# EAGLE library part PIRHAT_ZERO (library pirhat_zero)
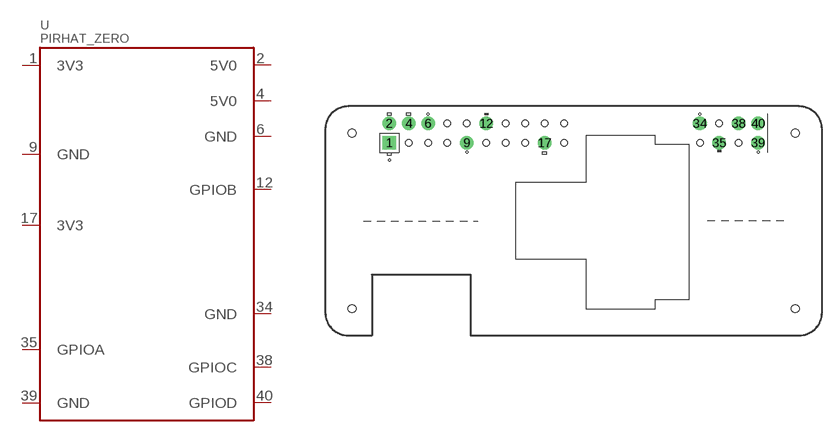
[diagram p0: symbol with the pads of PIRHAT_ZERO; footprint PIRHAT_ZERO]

Designator prefix -

## PIRHAT_ZERO  [PIRHAT_ZERO]
1  3V3  pwr
2  5V0  pwr
4  5V0  pwr
6  GND  sup
9  GND  sup
12  GPIOB
17  3V3  pwr
34  GND  sup
35  GPIOA
38  GPIOC
39  GND  sup
40  GPIOD

## Footprint PIRHAT_ZERO (pad centres in mm)
Raspberry Pi Zero W IR Hat, full outline with position of big connectors & drill holes
drill 1 pad 1.778 square: 1 8.37,25.23
drill 1 pad 1.778: 2 8.37,27.77; 4 10.91,27.77; 6 13.45,27.77; 9 18.53,25.23; 12 21.07,27.77; 17 28.69,25.23; 34 49.01,27.77; 35 51.55,25.23; 38 54.09,27.77; 39 56.63,25.23; 40 56.63,27.77
hole 1 at 3.5,3.5
hole 1 at 3.5,26.5
hole 1 at 61.5,3.5
hole 1 at 61.5,26.5
hole 0.85 at 54.09,25.23
hole 0.85 at 51.55,27.77
hole 0.85 at 31.23,25.23
hole 0.85 at 26.15,25.23
hole 0.85 at 15.99,27.77
hole 0.85 at 49.01,25.23
hole 0.85 at 23.61,25.23
hole 0.85 at 15.99,25.23
hole 0.85 at 13.45,25.23
hole 0.85 at 10.91,25.23
hole 0.85 at 21.07,25.23
hole 0.85 at 23.61,27.77
hole 0.85 at 28.69,27.77
hole 0.85 at 31.23,27.77
hole 0.85 at 26.15,27.77
hole 0.85 at 18.53,27.77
